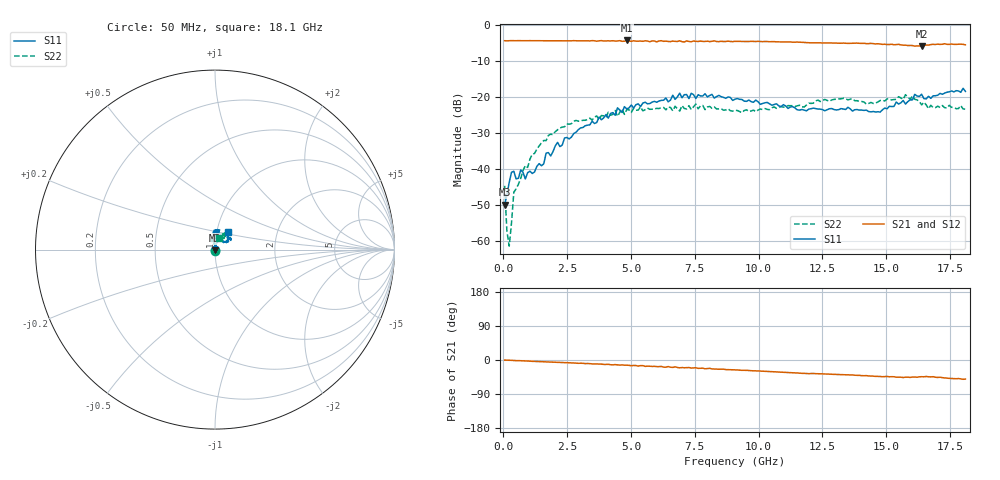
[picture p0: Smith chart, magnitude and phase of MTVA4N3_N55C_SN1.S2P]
! Network Analyzer HP8720D.06.14 Serial No. US36140669
! 11 May 2005  09:53:13
! Frequency  S11  S21  S12  S22
# HZ  S  DB R 50
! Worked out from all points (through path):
!   201 points, 50 MHz to 18.1 GHz, reference 50 ohm
!   highest |S21| = -4.28 dB at 4.833 GHz (marker M1); lowest = -5.9 dB at 16.39 GHz (marker M2)
!   group delay of S21, straight-line fit = 7.84 ps
!   lowest |S11| = -49.9 dB at 50 MHz (marker M3), VSWR 1.01, Z = 50.1 - j0.3 ohm
!   |S11| at or under -10 dB: start of sweep to end of sweep
!   |S22| runs from -61.4 to -19.3 dB; largest |S21 - S12| = 0.022
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5e7  -49.91 -69.5  -4.35 -0.3  -4.37 -0.6  -44.66 -98.1
1.4025e8  -47.24 -154.1  -4.38 -0.4  -4.39 -0.9  -57.34 23.4
2.305e8  -43.72 174.8  -4.36 -0.7  -4.34 -1.2  -61.44 -19.5
4.11e8  -40.63 178.5  -4.35 -1.3  -4.35 -1.7  -46.45 114.8
5.0125e8  -42.76 -179.1  -4.36 -1.6  -4.34 -1.9  -45.50 99.2
6.8175e8  -40.27 155.4  -4.34 -2.0  -4.35 -2.4  -42.60 113.1
8.6225e8  -42.77 144.9  -4.34 -2.5  -4.36 -2.9  -39.02 115.2
9.525e8  -41.01 138.6  -4.34 -2.7  -4.33 -3.2  -39.56 102.5
1.58425e9  -38.55 92.5  -4.36 -4.7  -4.36 -5.0  -32.07 98.4
1.76475e9  -35.44 102.3  -4.36 -5.1  -4.35 -5.5  -30.70 97.4
3.1185e9  -28.45 76.1  -4.37 -8.7  -4.39 -9.4  -26.46 110.5
4.83325e9  -23.30 80.1  -4.28 -13.6  -4.37 -14.8  -23.51 92.8
6.09675e9  -21.11 79.9  -4.42 -17.5  -4.37 -17.8  -23.19 90.2
6.909e9  -18.91 82.5  -4.36 -20.6  -4.48 -20.2  -23.90 80.1
7.54075e9  -20.42 80.8  -4.52 -20.5  -4.39 -22.4  -21.94 83.6
9.075e9  -20.61 92.6  -4.53 -26.1  -4.51 -26.5  -23.67 69.4
1.21435e10  -23.08 86.3  -4.94 -35.5  -4.90 -36.1  -21.69 69.2
1.476075e10  -24.18 41.5  -5.29 -43.4  -5.34 -44.3  -20.96 70.3
1.512175e10  -22.57 35.9  -5.41 -44.2  -5.28 -44.3  -20.57 67.7
1.57535e10  -21.95 35.5  -5.57 -45.3  -5.74 -46.4  -19.34 59.2
1.638525e10  -19.23 34.1  -5.89 -44.1  -5.71 -44.1  -22.19 52.3
1.81e10  -18.43 52.9  -5.48 -50.3  -5.52 -51.6  -23.38 70.7
